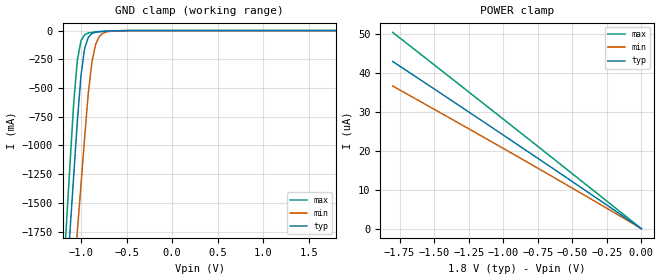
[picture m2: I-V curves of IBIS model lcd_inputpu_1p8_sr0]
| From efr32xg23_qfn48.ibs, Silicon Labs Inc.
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|   Model lcd_inputpu_1p8_sr0
[Model]  lcd_inputpu_1p8_sr0
Model_type Input
C_comp   1.6300pF   1.4000pF   2.7000pF
[Temperature Range]   25.0000   0.1250k   -40.0000
[Pullup Reference]   1.8000V   1.6200V   1.9800V
[Pulldown Reference]   0.0V   0.0V   0.0V
[POWER Clamp Reference]   1.8000V   1.6200V   1.9800V
[GND Clamp Reference]   0.0V   0.0V   0.0V
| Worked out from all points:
|   GND clamp passes 1 mA (typ) near -0.56 V on its own axis
[GND_clamp]
|Voltage   I(typ)   I(min)   I(max)
-1.8V     -9.867A    -9.569A    -10.32A
-1.2V     -2.688A    -3.389A    -2.224A
-1.16V    -2.211A    -2.978A    -1.687A
-1.12V    -1.735A    -2.567A    -1.152A
-1.08V    -1.26A     -2.157A    -630.4mA
-1.04V    -786.2mA   -1.747A    -256.2mA
-1V       -388.1mA   -1.338A    -87.65mA
-960mV    -155.8mA   -930mA     -35.81mA
-880mV    -25.09mA   -272.8mA   -16.36mA
-840mV    -13.97mA   -121.6mA   -10.53mA
-760mV    -7.874mA   -22.82mA   -6.602mA
1.8V      410.4pA    3.783uA    -5.116uA
[POWER_clamp]
|Voltage   I(typ)   I(min)   I(max)
-1.8V     42.99uA    36.68uA    50.46uA
-840mV    20.26uA    17.39uA    23.69uA
-420mV    10.18uA    8.771uA    11.88uA
0V        410.4pA    7.313nA    393.9pA
